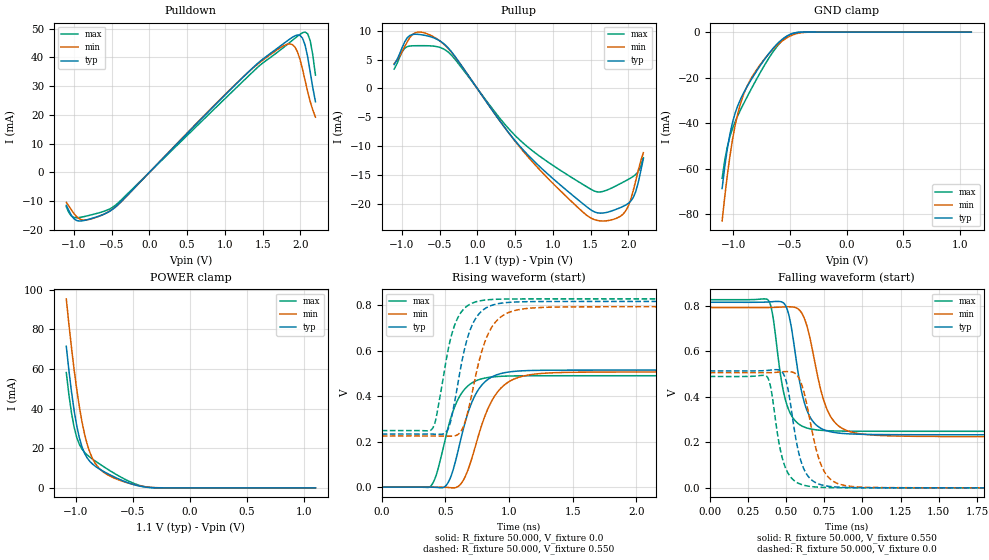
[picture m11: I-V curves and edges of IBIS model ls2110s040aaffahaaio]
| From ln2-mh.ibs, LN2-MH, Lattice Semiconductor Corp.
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|   Model ls2110s040aaffahaaio
[Model] ls2110s040aaffahaaio
| Clamp models do not include dynamic input termination. Please refer to
| the ls2110axxxaaffahaain model for input termination.
Model_type I/O
Polarity   Non-Inverting
Enable   Active-Low
Vinl =  0.200V
Vinh =  0.300V
Vmeas =  0.550V
Cref =  20.000pF
Rref =  50.000
Vref =  0.600V
C_comp   2.000pF   1.500pF   2.500pF
[Temperature Range]   25.000   0.125k   -40.000
[Voltage Range]   1.100V   1.070V   1.130V
[C Comp Corner]
C_comp   2.000pF   1.500pF   2.500pF
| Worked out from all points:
|   slope of the pulldown table from 0 to 0.165 V, typ, clamps not added: 36.9 ohm
|   slope of the pullup table from 0 to 0.165 V, typ, clamps not added: 52.6 ohm
|   GND clamp passes 1 mA (typ) near -0.50 V on its own axis
|   POWER clamp passes 1 mA (typ) near -0.45 V on its own axis
|   rising waveform, R_fixture 50.000, V_fixture 0.0: 20-80 % time 167ps typ, 199ps min, 154ps max; typ from 0 V to 0.515 V
|   rising waveform, R_fixture 50.000, V_fixture 0.550: 20-80 % time 136ps typ, 162ps min, 125ps max; typ from 0.233 V to 0.816 V
|   falling waveform, R_fixture 50.000, V_fixture 0.550: 20-80 % time 95.5ps typ, 123ps min, 82.8ps max; typ from 0.816 V to 0.233 V
|   falling waveform, R_fixture 50.000, V_fixture 0.0: 20-80 % time 86.1ps typ, 106ps min, 78.7ps max; typ from 0.515 V to 0 V
[Pulldown]
|Voltage   I(typ)   I(min)   I(max)
-1.1V     -11.44mA   -10.41mA   -11.96mA
-1.032V   -14.92mA   -13.01mA   -15.18mA
-896mV    -16.84mA   -16.44mA   -15.53mA
-488mV    -12.86mA   -12.79mA   -12.15mA
1.246V    33.22mA    33.26mA    31.81mA
1.824V    45.66mA    44.54mA    44.41mA
1.926V    47.43mA    43.65mA    46.57mA
2.028V    46.68mA    35.94mA    48.54mA
2.062V    44.32mA    32.03mA    48.79mA
2.13V     35mA       24.68mA    45.83mA
2.164V    29.56mA    21.75mA    40.94mA
2.2V      24.55mA    19.2mA     33.8mA
[Pullup]
|Voltage   I(typ)   I(min)   I(max)
-1.1V     4.135mA    4.293mA    3.355mA
-996mV    7.03mA     6.335mA    6.318mA
-894mV    9.159mA    8.78mA     7.344mA
-758mV    9.324mA    9.762mA    7.4mA
-486mV    8.157mA    8.129mA    7.064mA
-316mV    5.917mA    5.851mA    5.381mA
568mV     -10.04mA   -10.2mA    -8.966mA
1.554V    -21.35mA   -22.68mA   -17.75mA
1.792V    -21.12mA   -22.67mA   -17.13mA
1.962V    -20.18mA   -21.24mA   -15.99mA
2.098V    -17.86mA   -15.98mA   -14.88mA
2.2V      -12.11mA   -11.1mA    -11.96mA
[GND_clamp]
|Voltage   I(typ)   I(min)   I(max)
-1.1V     -68.65mA   -82.91mA   -64.16mA
-1.054V   -51.26mA   -62.87mA   -50.37mA
-1.008V   -39.63mA   -47.13mA   -42.26mA
-962mV    -32.34mA   -35.82mA   -36.73mA
-916mV    -27.28mA   -28.13mA   -32.02mA
-847mV    -21.22mA   -20.63mA   -25.4mA
-778mV    -15.81mA   -15.27mA   -19.09mA
-663mV    -7.926mA   -8.201mA   -9.607mA
-571mV    -3.246mA   -3.982mA   -3.828mA
-502mV    -1.097mA   -1.819mA   -1.164mA
-410mV    -96.97uA   -374.9uA   -57.53uA
1.1V      0A         0A         0A
[POWER_clamp]
|Voltage   I(typ)   I(min)   I(max)
-1.085V   71.41mA    95.35mA    58.18mA
-1.062V   59.23mA    82.55mA    46.99mA
-1.039V   48.36mA    70.56mA    37.71mA
-1.016V   38.97mA    59.53mA    30.53mA
-970mV    25.17mA    40.76mA    21.88mA
-924mV    17.37mA    26.93mA    17.87mA
-901mV    15.03mA    21.86mA    16.59mA
-855mV    12.01mA    14.79mA    14.5mA
-763mV    8.448mA    8.108mA    10.89mA
-533mV    2.369mA    2.267mA    3.272mA
-349mV    143.9uA    291.4uA    171.3uA
1.1V      0A         0A         0A
[Ramp]
| variable   typ   min   max
dV/dt_r   0.309/0.167n   0.304/0.199n   0.294/0.154n
dV/dt_f   0.379/0.106n   0.371/0.143n   0.381/87.930p
R_load = 50.000
[Rising Waveform]
R_fixture= 50.000
V_fixture= 0.0
V_fixture_min= 0.0
V_fixture_max= 0.0
|time   V(typ)   V(min)   V(max)
0s        1.068uV    5.74uV     488.6nV
390ps     -100.3uV   59.18uV    8.073mV
512ps     12.34mV    -1.152mV   241.4mV
603ps     168.7mV    4.393mV    390.6mV
680ps     331.5mV    80.56mV    446.8mV
766ps     434.5mV    239.3mV    473.2mV
883ps     489.5mV    397.4mV    485.3mV
1.036ns   508.8mV    474.6mV    489mV
1.726ns   514.5mV    506.1mV    489.9mV
10ns      514.6mV    506.5mV    490mV
[Rising Waveform]
R_fixture= 50.000
V_fixture= 0.550
V_fixture_min= 0.534
V_fixture_max= 0.568
|time   V(typ)   V(min)   V(max)
0s        233.5mV    224.9mV    248.7mV
390ps     233.4mV    225mV      252.5mV
425ps     232.8mV    225mV      299.3mV
509ps     244.8mV    224.2mV    567.8mV
639ps     579mV      263.2mV    780mV
715ps     718.8mV    429.3mV    810.1mV
820ps     788.2mV    653.8mV    823.1mV
969ps     810.9mV    760.7mV    827mV
1.289ns   816.2mV    790.8mV    827.7mV
10ns      816.5mV    793.4mV    827.8mV
[Falling Waveform]
R_fixture= 50.000
V_fixture= 0.550
V_fixture_min= 0.534
V_fixture_max= 0.568
|time   V(typ)   V(min)   V(max)
0s        816.4mV    793.4mV    827.8mV
387ps     817.8mV    793.5mV    822.3mV
412ps     819.1mV    793.8mV    762.3mV
490ps     808.8mV    796.3mV    402.9mV
527ps     734.1mV    796.6mV    329mV
618ps     378.9mV    748.2mV    267.7mV
723ps     263.9mV    442.6mV    253.4mV
853ps     240.4mV    267.8mV    249.9mV
1.153ns   234.2mV    229.3mV    248.8mV
10ns      233.5mV    224.9mV    248.7mV
[Falling Waveform]
R_fixture= 50.000
V_fixture= 0.0
V_fixture_min= 0.0
V_fixture_max= 0.0
|time   V(typ)   V(min)   V(max)
0s        514.6mV    506.5mV    489.9mV
377ps     516.5mV    506.7mV    488mV
401ps     518.3mV    507.1mV    437.3mV
451ps     519.1mV    509.2mV    208.2mV
490ps     491.4mV    511.3mV    99.23mV
564ps     217.2mV    501mV      26.58mV
642ps     53.04mV    346.6mV    7.83mV
723ps     14.73mV    112.3mV    2.569mV
813ps     4.489mV    26.9mV     889.8uV
10ns      1.053uV    5.719uV    475nV
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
